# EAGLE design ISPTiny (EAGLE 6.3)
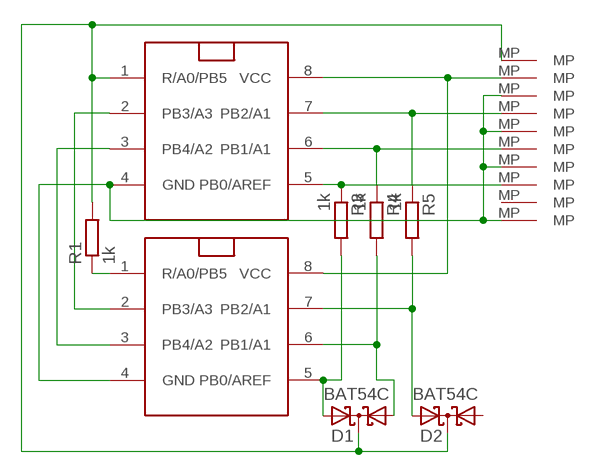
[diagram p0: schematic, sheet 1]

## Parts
BRD  Socket  ATTINY85  [DIL08]
D1  BAT54C  [SOT23]
D2  BAT54C  [SOT23]
MC  ATTINY85  [DIL08]
R1  1k  R-EU_R0603  [R0603]
R3  1k  R-EU_R0603  [R0603]
R4  1k  R-EU_R0603  [R0603]
R5  1k  R-EU_R0603  [R0603]
U$1  SMD-RM1.27  [SMD-RM1.27]
U$2  SMD-RM1.27  [SMD-RM1.27]
U$3  SMD-RM1.27  [SMD-RM1.27]
U$4  SMD-RM1.27  [SMD-RM1.27]
U$5  SMD-RM1.27  [SMD-RM1.27]
U$6  SMD-RM1.27  [SMD-RM1.27]
U$7  SMD-RM1.27  [SMD-RM1.27]
U$8  SMD-RM1.27  [SMD-RM1.27]
U$9  SMD-RM1.27  [SMD-RM1.27]
U$10  SMD-RM1.27  [SMD-RM1.27]

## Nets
GND: BRD.4(GND) MC.4(GND) U$2.MP U$4.MP U$7.MP U$9.MP
MISO: MC.6(PB1/A1) R4.1 U$6.MP
MOSI: MC.5(PB0/AREF) R3.1 U$8.MP
N$1: BRD.1(R/A0/PB5) R1.1
N$6: BRD.5(PB0/AREF) D1.2(A2) R3.2
N$7: BRD.6(PB1/A1) D1.1(A1) R4.2
N$8: BRD.7(PB2/A1) D2.2(A2) R5.2
N$12: BRD.2(PB3/A3) MC.2(PB3/A3)
N$20: BRD.3(PB4/A2) MC.3(PB4/A2)
RST: D1.3(CC) D2.3(CC) MC.1(R/A0/PB5) R1.2 U$5.MP
SCK: MC.7(PB2/A1) R5.1 U$3.MP
VTG: BRD.8(VCC) MC.8(VCC) U$1.MP
Unconnected: D2.1(A1) U$10.MP

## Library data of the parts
BRD MC = atmel:ATTINY85
D1 D2 = diode:BAT54C: Schottky Diodes Source: Fairchild .. BAT54.pdf
R1 R3-R5 = rcl:R-EU_: RESISTOR, European symbol
U$1-U$10 = solpad:SMD-RM1.27

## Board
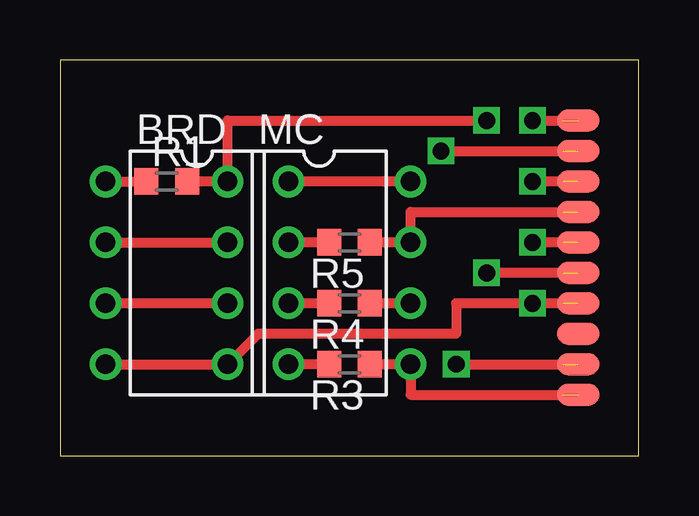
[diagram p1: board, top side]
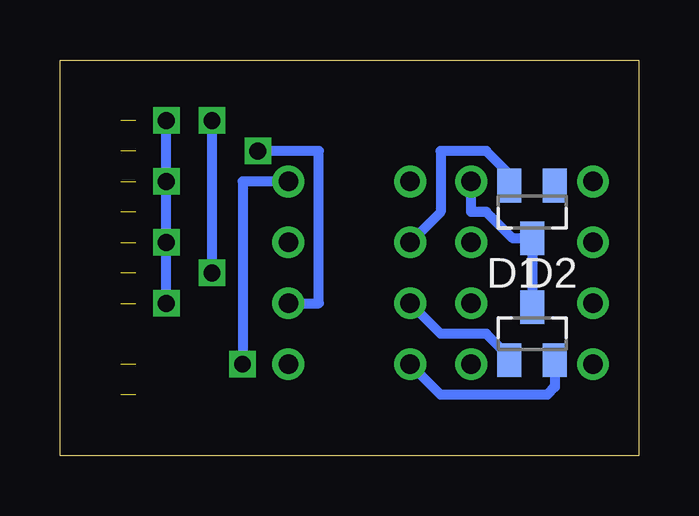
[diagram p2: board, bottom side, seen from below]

Size 24.12 x 16.5 mm. Coordinates in mm from the lower left corner, seen from the top.
Outline: 0,0 24.12,0 24.12,16.5 0,16.5 0,0
Copper layers (1*16): Top 0.035mm / dielectric 1.5mm / Bottom 0.035mm
Design rules "default": minimum track width 10mil, minimum drill 24mil, track to track 8mil, track to pad 8mil, pad to pad 8mil, via to via 8mil, smd to smd 8mil, copper to edge 40mil, drill to drill 8mil, minimum pad ring 10mil, minimum via ring 8mil, stop-mask expansion 4mil, vias tented up to drill 0mil, thermal gap 10mil

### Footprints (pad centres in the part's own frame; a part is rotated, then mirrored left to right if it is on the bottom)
DIL08 = drill 0.813: 1 -3.81,-3.81; 2 -1.27,-3.81; 3 1.27,-3.81; 4 3.81,-3.81; 5 3.81,3.81; 6 1.27,3.81; 7 -1.27,3.81; 8 -3.81,3.81
SOT23 = smd 1 x 1.4: 1 -0.95,-1.1; 2 0.95,-1.1; 3 0,1.1
R0603 = smd 1 x 1.1: 1 -0.85,0; 2 0.85,0
SMD-RM1.27 = smd 1.778 x 0.914: MP 0,0

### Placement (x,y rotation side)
BRD  5.71,7.62 270 top
D1  4.45,5.08 0 bottom
D2  4.45,10.16 180 bottom
MC  10.79,7.62 270 top
R1  4.45,11.43 0 top
R3  12.06,3.81 180 top
R4  12.06,6.35 180 top
R5  12.06,8.89 180 top
U$1  21.59,3.81 0 top
U$2  21.59,6.35 0 top
U$3  21.59,10.16 0 top
U$4  21.59,8.89 0 top
U$5  21.59,7.62 0 top
U$6  21.59,12.7 0 top
U$7  21.59,11.43 0 top
U$8  21.59,2.54 0 top
U$9  21.59,13.97 0 top
U$10  21.59,5.08 0 top

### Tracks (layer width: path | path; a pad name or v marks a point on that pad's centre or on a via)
GND  (via drill 0.7)  (4 unrouted)
  Top 0.406: 20.95,6.35 v19.68,6.35 16.51,6.35 16.51,5.08 8.26,5.08 MC.4 BRD.4 | v19.68,13.97 20.95,13.97 | 20.95,8.89 v19.68,8.89 | 20.95,11.43 v19.68,11.43
  Bottom 0.406: v19.68,6.35 v19.68,8.89 v19.68,11.43 v19.68,13.97
MISO  (via drill 0.7)  (1 unrouted)
  Top 0.406: v15.88,12.7 20.95,12.7 | MC.6 R4.1
  Bottom 0.406: MC.6 13.34,6.35 13.34,12.7 v15.88,12.7
MOSI  (1 unrouted)
  Top 0.406: R3.1 MC.5 14.61,2.54 20.95,2.54
N$1
  Top 0.406: BRD.1 R1.1
N$6
  Top 0.406: R3.2 BRD.5
  Bottom 0.406: D1.2 3.5,2.85 3.81,2.54 8.26,2.54 BRD.5
N$7
  Top 0.406: R4.2 BRD.6
  Bottom 0.406: D1.1 5.39,4.12 6.35,5.08 8.26,5.08 BRD.6
N$8
  Top 0.406: R5.2 BRD.7
  Bottom 0.406: D2.2 5.39,11.74 6.35,12.7 8.26,12.7 8.26,10.16 BRD.7
N$12
  Top 0.406: BRD.2 MC.2
N$20
  Top 0.406: MC.3 BRD.3
RST  (via drill 0.7)  (1 unrouted)
  Top 0.406: R1.2 MC.1 6.99,13.97 v17.78,13.97 | 20.95,7.62 v17.78,7.62
  Bottom 0.406: v17.78,7.62 v17.78,13.97 | MC.1 6.99,10.16 6.35,10.16 5.25,9.06 D2.3 D1.3
SCK  (1 unrouted)
  Top 0.406: R5.1 MC.7 14.61,10.16 20.95,10.16
VTG  (via drill 0.7)  (1 unrouted)
  Top 0.406: v16.51,3.81 20.95,3.81 | MC.8 BRD.8
  Bottom 0.406: MC.8 16.51,11.43 v16.51,3.81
